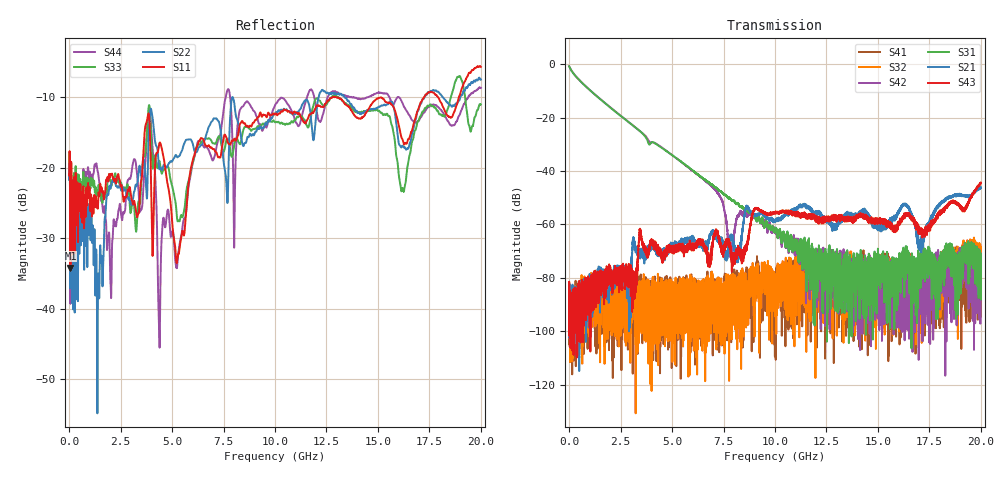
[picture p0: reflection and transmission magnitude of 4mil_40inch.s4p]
!Agilent Technologies,N5230A,US43500443,A.06.04.32
!Agilent N5230A: A.06.04.32
!Date: Wednesday, December 12, 2012 17:10:51
!Correction: S11(Full 4 Port(1,2,3,4)) S12(Full 4 Port(1,2,3,4)) S13(Full 4 Port(1,2,3,4)) S14(Full 4 Port(1,2,3,4)) S21(Full 4 Port(1,2,3,4)) S22(Full 4 Port(1,2,3,4)) S23(Full 4 Port(1,2,3,4)) S24(Full 4 Port(1,2,3,4)) S31(Full 4 Port(1,2,3,4)) S32(Full 4 Port(1,2,3,4)) S33(Full 4 Port(1,2,3,4)) S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
!S4P File: Measurements: <S11,S12,S13,S14>, <S21,S22,S23,S24>, <S31,S32,S33,S34>, <S41,S42,S43,S44>:
# Hz S  dB  R 50
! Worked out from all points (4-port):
!   10000 points, 1 MHz to 20 GHz, reference 50 ohm
!   strongest paths, dB at 1 MHz, 5.001 GHz, 10 GHz, 15 GHz, 20 GHz:
!     S43: -87.4, -70.7, -55.6, -58.6, -44.3
!     S21: -87.6, -68.2, -58.4, -62.2, -46.2
!     S31: -0.8, -34.0, -62.9, -75.3, -73.0
!     S42: -0.8, -34.0, -62.6, -76.4, -85.0
!     S32: -81.8, -92.5, -80.1, -81.7, -71.6
!     S41: -83.4, -92.0, -84.5, -86.9, -86.0
!   lowest |S11| = -34.2 dB at 65 MHz (marker M1), VSWR 1.04, Z = 51.9 - j0.645 ohm
!   |S11| at or under -10 dB: start of sweep to 12.79 GHz; 12.98 GHz to 15.14 GHz (2.155 GHz wide, 15.3 % of centre); 15.14 GHz to 17.24 GHz (2.099 GHz wide, 13 % of centre)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
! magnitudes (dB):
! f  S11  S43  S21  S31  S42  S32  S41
! 1 MHz  -21.1  -87.4  -87.6  -0.8  -0.8  -81.8  -83.4
! 65 MHz  -34.2  -94.6  -90.3  -1.8  -1.7  -94.9  -91.2
! 3.901 GHz  -13.3  -68.1  -69.3  -30.1  -29.0  -87.1  -84.8
! 4.387 GHz  -16.5  -69.4  -70.7  -30.8  -30.5  -90.6  -93.1
! 7.839 GHz  -16.7  -69.3  -64.9  -50.4  -70.9  -87.9  -79.4
! 13.16 GHz  -10.2  -57.2  -58.7  -77.6  -74.4  -77.0  -87.7
! 20 GHz  -5.7  -44.3  -46.2  -73.0  -85.0  -71.6  -86.0
